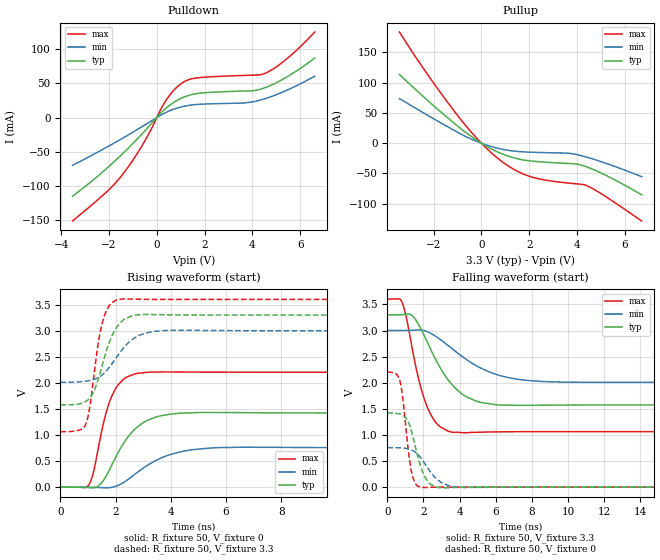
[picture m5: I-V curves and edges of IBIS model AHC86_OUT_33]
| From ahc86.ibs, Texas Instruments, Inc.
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[Model]   AHC86_OUT_33
Model_type  Output
|Vref =   0
|Rref =   1000
Cref =   50
Vmeas =   1.65
| variable   typ   min   max
C_comp   12.49pF   10.99pF   14.17pF
| C_pullup   12.14pF   10.99pF   13.48pF
| C_pulldown   12.84pF   11.21pF   14.17pF
[Temperature Range]   40   100   -40
| Ambient temperature   25   85   -40
[Voltage range]   3.3   3   3.6
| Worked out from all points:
|   slope of the pulldown table from 0 to 0.495 V, typ, clamps not added: 29.4 ohm
|   slope of the pullup table from 0 to 0.495 V, typ, clamps not added: 44.5 ohm
|   rising waveform, R_fixture 50, V_fixture 0: 20-80 % time 1.02ns typ, 1.41ns min, 616ps max; typ from 0 V to 1.42 V
|   falling waveform, R_fixture 50, V_fixture 3.3: 20-80 % time 1.72ns typ, 2.61ns min, 1.02ns max; typ from 3.3 V to 1.58 V
|   rising waveform, R_fixture 50, V_fixture 3.3: 20-80 % time 641ps typ, 907ps min, 418ps max; typ from 1.58 V to 3.3 V
|   falling waveform, R_fixture 50, V_fixture 0: 20-80 % time 681ps typ, 1.01ns min, 428ps max; typ from 1.42 V to 0 V
[Pulldown]
| AHC86_OUT_33
|   Voltage   I(typ)   I(min)   I(max)
-3.525V   -115.6mA   -70.3mA    -152mA
-2.09V    -74.61mA   -43.5mA    -108.9mA
-1.505V   -55.66mA   -31.95mA   -86.88mA
-550mV    -21.61mA   -11.89mA   -37.48mA
355mV     12.74mA    6.975mA    23.52mA
955mV     27.12mA    14.92mA    47.99mA
1.225V    31.15mA    17.11mA    54.02mA
1.63V     34.84mA    19.02mA    57.91mA
3.605V    38.8mA     21.23mA    61.73mA
4.52V     43.69mA    27.57mA    64.75mA
5.475V    60.21mA    40.57mA    87.17mA
6.61V     87.31mA    60.67mA    125.5mA
[Pullup]
| AHC86_OUT_33
|   Voltage   I(typ)   I(min)   I(max)
-3.43V    113.4mA    73.61mA    183.6mA
-2.11V    65.76mA    42.94mA    105.4mA
-830mV    22.9mA     14.53mA    37.35mA
105mV     -2.578mA   -1.53mA    -4.254mA
800mV     -16.66mA   -9.429mA   -28.58mA
1.435V    -25.04mA   -13.4mA    -44.88mA
2.135V    -29.66mA   -14.98mA   -56.22mA
3.61V     -33.44mA   -16.56mA   -65.78mA
4.205V    -36.54mA   -20.91mA   -68mA
4.47V     -40.15mA   -23.81mA   -71.19mA
4.9V      -47.28mA   -29.07mA   -80.65mA
6.705V    -85.23mA   -55.27mA   -128.5mA
[Ramp]
| AHC86_OUT_33
| variable   typ   min   max
dV/dt_r   0.87/1.07E-09   0.47/1.52E-09   1.33/6.28E-10
dV/dt_f   1.05/1.76E-09   0.60/2.67E-09   1.53/1.07E-09
R_load = 50
[Rising Waveform]
| AHC86_OUT_33
R_fixture =   50
C_fixture =   0
L_fixture =   0
V_fixture =   0
V_fixture_min = 0
V_fixture_max = 0
|   Time   V(typ)   V(min)   V(max)
0s        -94.41uV   -113.1uV   -57.67uV
1.01ns    -7.936mV   -1.922mV   30.53mV
1.19ns    -11.74mV   -3.339mV   273.3mV
1.46ns    64.54mV    -9.034mV   984.8mV
1.955ns   522.8mV    9.124mV    1.847V
2.4ns     926.9mV    128.9mV    2.11V
3.16ns    1.282V     420.7mV    2.203V
4.505ns   1.422V     694.1mV    2.208V
6.48ns    1.43V      765.4mV    2.204V
50ns      1.421V     756.2mV    2.202V
[Falling Waveform]
| AHC86_OUT_33
R_fixture =   50
C_fixture =   0
L_fixture =   0
V_fixture =   3.3
V_fixture_min = 3
V_fixture_max = 3.6
|   Time   V(typ)   V(min)   V(max)
0s        3.3V       3V         3.6V
795ps     3.304V     3.001V     3.556V
1.05ns    3.311V     3.002V     3.253V
1.42ns    3.271V     3.005V     2.577V
2.17ns    2.807V     2.985V     1.569V
2.77ns    2.384V     2.868V     1.203V
3.585ns   1.962V     2.652V     1.053V
5.225ns   1.619V     2.271V     1.052V
8.74ns    1.569V     2.021V     1.062V
50ns      1.577V     2.01V      1.064V
[Rising Waveform]
| AHC86_OUT_33
R_fixture =   50
C_fixture =   0
L_fixture =   0
V_fixture =   3.3
V_fixture_min = 3
V_fixture_max = 3.6
|   Time   V(typ)   V(min)   V(max)
0s        1.577V     2.01V      1.064V
910ps     1.641V     2.032V     1.199V
1.045ns   1.698V     2.045V     1.48V
1.22ns    1.85V      2.069V     2.163V
1.535ns   2.378V     2.162V     3.184V
1.795ns   2.808V     2.313V     3.499V
2.125ns   3.123V     2.558V     3.601V
2.85ns    3.305V     2.909V     3.603V
4.005ns   3.304V     3.009V     3.599V
50ns      3.3V       3V         3.6V
[Falling Waveform]
| AHC86_OUT_33
R_fixture =   50
C_fixture =   0
L_fixture =   0
V_fixture =   0
V_fixture_min = 0
V_fixture_max = 0
|   Time   V(typ)   V(min)   V(max)
0s        1.421V     756.2mV    2.202V
690ps     1.401V     752.9mV    2.044V
840ps     1.378V     749.2mV    1.748V
1.155ns   1.252V     730.8mV    721.5mV
1.33ns    1.08V      711mV      309.4mV
1.57ns    744.6mV    663.1mV    63.57mV
1.89ns    348.8mV    542mV      -7.039mV
2.645ns   7.554mV    185.2mV    -767.7uV
4.27ns    -2.499mV   -6.121mV   -122.2uV
50ns      -94.38uV   -113uV     -57.67uV
